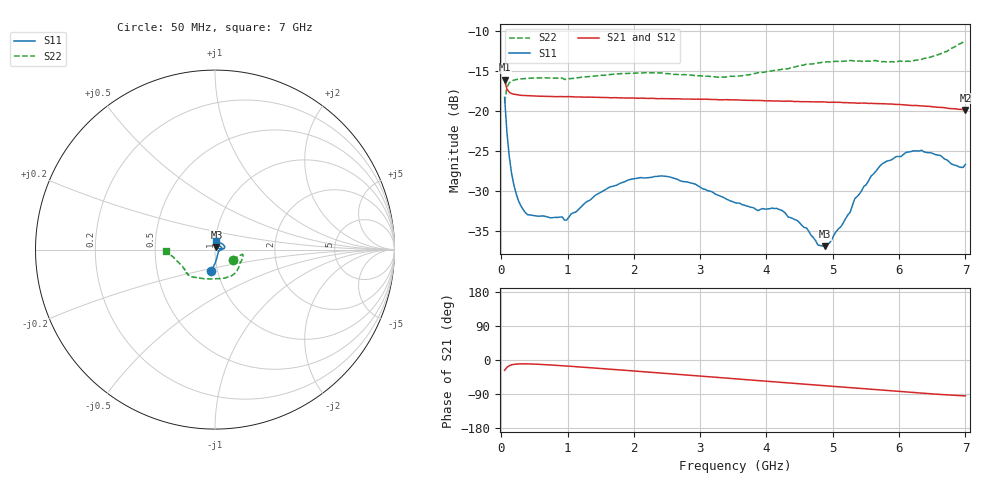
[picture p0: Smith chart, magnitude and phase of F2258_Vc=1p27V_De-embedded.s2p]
! Integrated Device Technology
! Corporate Headquarters
! 6024 Silver Creek Valley Road
! San Jose, CA 95138  USA
! Phone:  1-408-284-8200
! Toll Free:  1-800-223-1366
! Webpage:  http://www.idt.com/
! Timing and RF Division
! 515 Groton Road, Suite 102
! Westford, MA 01886-6024
! Device:  F2258
! Description: Voltage Variable RF Attenuator
! Frequency:  50.0 -  6000.00 MHz
! Package:  3x3 mm Thin QFN Plastic Package: 16 pin
! Ports:  2 RF, 2 DC
!  Pin  1  = NC
!  Pin  2  = NC
!  Pin  3  = RF2  = Port 2
!  Pin  4  = GND
!  Pin  5  = Vdd
!  Pin  6  = NC
!  Pin  7  = VCTRL
!  Pin  8  = NC
!  Pin  9  = GND
!  Pin 10  = RF1  = Port 1
!  Pin 11  = NC
!  Pin 12  = NC
!  Pin 13  = NC
!  Pin 14  = NC
!  Pin 15  = NC
!  Pin 16  = NC
! Vcntrl:  1.270 Volts
! Vdd:  +3.300 Volts
! Current:  1.162 mA
! Data:  The device was measured on a the F2258 evaluation board which has
!  individual transmission lines to the RF pins.  Data was collected
!  using a calibrated network analyzer.  The evaluation board was
!  de-embedded using a TRL calibration technique.
!  The reference plane is the edge of the package pin.
! Misc:  SN 10
!  Action Tracker AT0285
! Date Measured:  2014-12-10
! Date:  2016-01-13  MJV
! Note:
!  Integrated Device Technology supplies this data as a sample of measured
!  data at the package pin for this product.  Your particular data for this
!  product may vary.
!  Data was taken at 25 degrees C.
!  Integrated Device Technology reserves the right to change this data at anytime.
!Freq_(GHz)  S11M_(dB)  S11P_(deg)  S21M_(dB)  S21P_(deg)  S12M_(dB)  S12P_(deg)  S22M_(dB)  S22P_(deg)
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# GHz S dB R 50
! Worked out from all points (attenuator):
!   201 points, 50 MHz to 7 GHz, reference 50 ohm
!   highest |S21| = -16.11 dB at 50 MHz (marker M1); lowest = -19.9 dB at 7 GHz (marker M2)
!   lowest |S11| = -36.9 dB at 4.88 GHz (marker M3), VSWR 1.03, Z = 50.8 + j1.2 ohm
!   |S11| at or under -10 dB: start of sweep to end of sweep
!   |S22| runs from -19.0 to -11.2 dB; largest |S21 - S12| = 0.0012
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0.05  -18.31 -99.5  -16.11 -27.4  -16.05 -27.3  -18.96 -29.3
0.08475  -22.68 -88.8  -17.28 -19.3  -17.23 -19.3  -17.08 -14.3
0.15425  -27.76 -73.1  -17.84 -13.0  -17.82 -12.9  -16.30 -10.2
0.2585  -31.19 -54.8  -18.01 -10.4  -18.04 -10.4  -16.05 -10.1
0.36275  -32.69 -41.5  -18.10 -10.1  -18.09 -10.1  -15.96 -11.9
0.98825  -33.62 -20.1  -18.23 -15.9  -18.27 -15.9  -16.06 -27.2
1.2315  -31.75 -11.8  -18.28 -18.9  -18.34 -18.9  -15.78 -32.8
1.6485  -29.46 -4.3  -18.37 -24.4  -18.39 -24.3  -15.47 -42.2
2.37825  -28.14 12.0  -18.49 -33.9  -18.51 -33.9  -15.26 -58.5
2.8995  -29.07 29.5  -18.55 -40.9  -18.57 -40.9  -15.57 -72.7
3.525  -31.45 62.9  -18.63 -49.5  -18.67 -49.5  -15.69 -96.0
3.8725  -32.45 86.1  -18.70 -54.3  -18.74 -54.2  -15.24 -109.3
4.22  -32.38 96.0  -18.79 -59.0  -18.82 -59.0  -14.84 -119.5
4.7065  -35.80 78.9  -18.87 -65.5  -18.89 -65.5  -14.13 -129.5
4.88025  -36.88 55.7  -18.89 -67.9  -18.93 -67.8  -13.89 -131.8
5.1235  -34.44 24.9  -18.94 -71.1  -18.97 -71.0  -13.84 -134.9
5.332  -30.96 9.8  -19.01 -73.9  -19.07 -73.7  -13.81 -136.9
5.57525  -28.16 5.6  -19.06 -77.0  -19.10 -76.9  -13.82 -140.6
5.85325  -26.20 7.3  -19.15 -80.8  -19.18 -80.8  -13.88 -145.3
6.33975  -24.92 18.3  -19.39 -87.4  -19.42 -87.4  -13.57 -157.4
6.9305  -27.05 72.8  -19.81 -94.1  -19.86 -93.9  -11.58 -175.8
7  -26.67 84.6  -19.88 -94.5  -19.90 -94.5  -11.22 -178.2
